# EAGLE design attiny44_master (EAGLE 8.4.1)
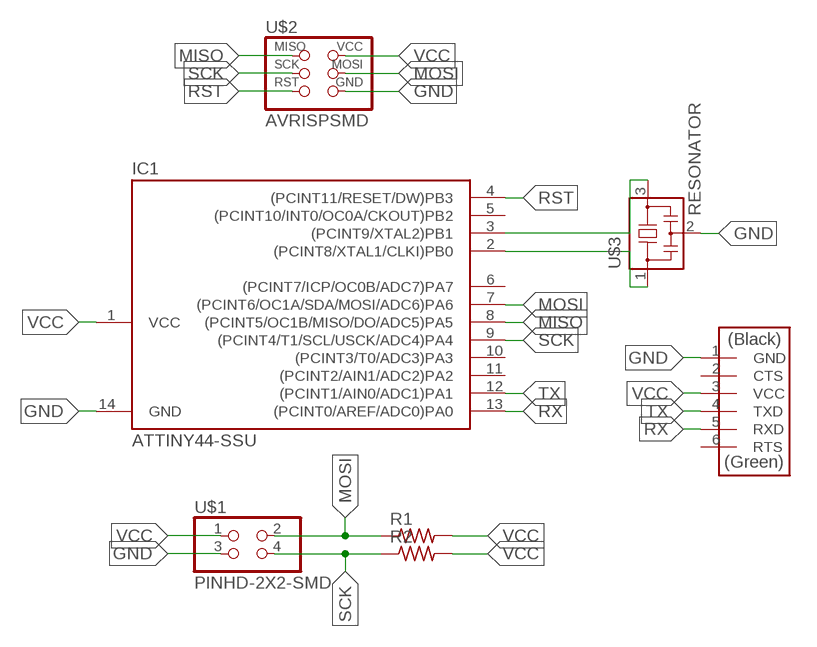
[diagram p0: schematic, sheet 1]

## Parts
IC1  ATTINY44-SSU  [SOIC14]
R1  RES-US1206FAB  [R1206FAB]
R2  RES-US1206FAB  [R1206FAB]
U$1  PINHD-2X2-SMD  [2X02SMD]
U$2  AVRISPSMD  [2X03SMD]
U$3  RESONATOR  [EFOBM]
U$4  FTDI-SMD-HEADER  [1X06SMD]

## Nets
GND: IC1.14(GND) U$1.3 U$2.6(GND) U$3.2 U$4.1(GND)
MISO: IC1.8((PCINT5/OC1B/MISO/DO/ADC5)PA5) U$2.1(MISO)
MOSI: IC1.7((PCINT6/OC1A/SDA/MOSI/ADC6)PA6) R1.1 U$1.2 U$2.4(MOSI)
N$5: IC1.3((PCINT9/XTAL2)PB1) U$3.3
N$6: IC1.2((PCINT8/XTAL1/CLKI)PB0) U$3.1
RST: IC1.4((PCINT11/RESET/DW)PB3) U$2.5(RST)
RX: IC1.13((PCINT0/AREF/ADC0)PA0) U$4.5(RXD)
SCK: IC1.9((PCINT4/T1/SCL/USCK/ADC4)PA4) R2.1 U$1.4 U$2.3(SCK)
TX: IC1.12((PCINT1/AIN0/ADC1)PA1) U$4.4(TXD)
VCC: IC1.1(VCC) R1.2 R2.2 U$1.1 U$2.2(VCC) U$4.3(VCC)
Unconnected: IC1.5((PCINT10/INT0/OC0A/CKOUT)PB2) IC1.6((PCINT7/ICP/OC0B/ADC7)PA7) IC1.10((PCINT3/T0/ADC3)PA3) IC1.11((PCINT2/AIN1/ADC2)PA2) U$4.2(CTS) U$4.6(RTS)

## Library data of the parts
IC1 = fab:ATTINY44
R1 R2 = fab:RES-US: Resistor (US Symbol)
U$1 = fab:PINHD-2X2-SMD
U$2 = fab:AVRISP
U$3 = fab:RESONATOR
U$4 = fab:FTDI-SMD-HEADER

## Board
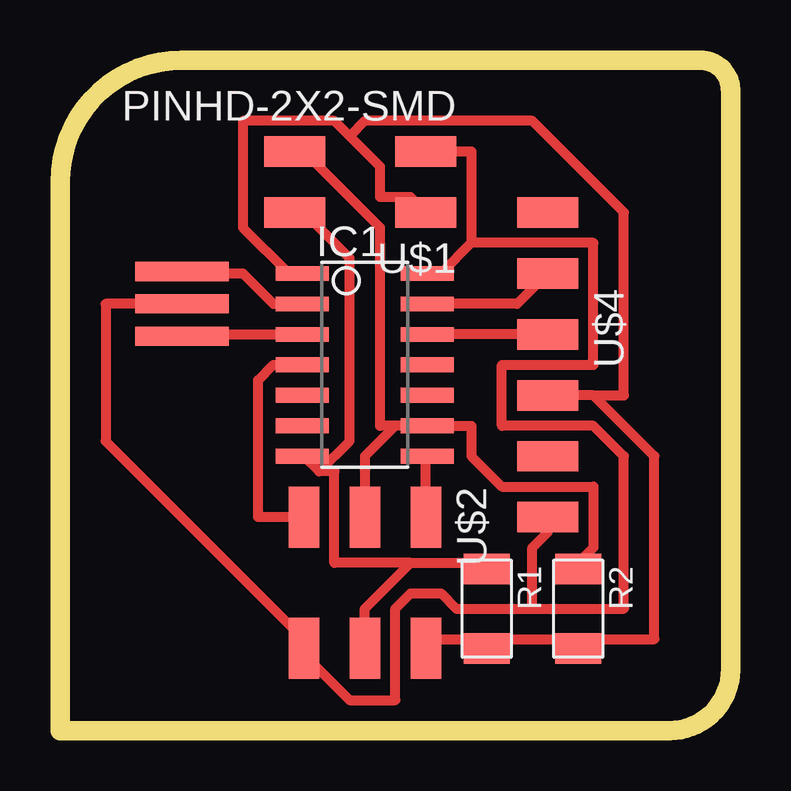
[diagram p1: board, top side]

Size 27.94 x 27.94 mm. Coordinates in mm from the lower left corner, seen from the top.
Outline: 0,22.86 arc-90 5.08,27.94 26.67,27.94 arc-90 27.94,26.67 27.94,2.54 arc-90 25.4,0 0,0 0,22.86
Copper layers (1*16): Top 0.035mm / dielectric 1.5mm / Bottom 0.035mm
Design rules "default *": minimum track width 16mil, minimum drill 0.35mm, track to track 16mil, track to pad 16mil, pad to pad 16mil, via to via 16mil, smd to smd 16mil, copper to edge 16mil, drill to drill 16mil, minimum pad ring 10mil, minimum via ring 8mil, stop-mask expansion 4mil, vias tented up to drill 0mil, thermal gap 10mil

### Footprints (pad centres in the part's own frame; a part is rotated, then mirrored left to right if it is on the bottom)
SOIC14 = smd 0.61 x 2.21: 1 -3.81,-2.603; 2 -2.54,-2.603; 3 -1.27,-2.603; 4 0,-2.603; 5 1.27,-2.603; 6 2.54,-2.603; 7 3.81,-2.603; 8 3.81,2.603; 9 2.54,2.603; 10 1.27,2.603; 11 0,2.603; 12 -1.27,2.603; 13 -2.54,2.603; 14 -3.81,2.603
R1206FAB = smd 1.27 x 1.905: 1 -1.651,0; 2 1.651,0
2X02SMD = smd 2.54 x 1.27: 1 -2.54,1.27; 2 2.92,1.27; 3 -2.54,-1.27; 4 2.92,-1.27
2X03SMD = smd 2.54 x 1.27: 1 -2.54,2.54; 2 2.92,2.54; 3 -2.54,0; 4 2.92,0; 5 -2.54,-2.54; 6 2.92,-2.54
EFOBM = smd 0.8 x 3.9: 1 -1.35,0; 2 0,0; 3 1.35,0
1X06SMD = smd 2.54 x 1.27: 1 0,6.35; 2 0,3.81; 3 0,1.27; 4 0,-1.27; 5 0,-3.81; 6 0,-6.35

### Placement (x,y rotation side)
IC1  12.7,15.24 270 top
R1  17.78,5.08 270 top
R2  21.59,5.08 270 top
U$1  12.7,22.86 180 top
U$2  12.7,6.35 270 top
U$3  5.08,17.78 270 top
U$4  20.32,15.24 180 top

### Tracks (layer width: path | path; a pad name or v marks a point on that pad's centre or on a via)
GND
  Top 0.406: 17.14,20.32 15.88,19.05 IC1.14 | 17.14,20.32 17.14,24.13 U$1.3 | U$3.2 1.9,17.78 1.9,12.07 10.16,3.81 U$2.6 10.16,3.18 12.06,1.27 13.97,1.27 13.97,5.08 14.6,5.71 15.88,5.71 16.51,5.08 19.69,5.08 | U$4.1 20.32,8.25 19.69,7.62 19.69,5.08 | 17.14,20.32 22.23,20.32 22.23,15.24 18.41,15.24 18.41,12.7 22.23,12.7 23.49,11.43 23.49,5.08 19.69,5.08
MISO
  Top 0.406: U$2.1 15.24,11.43 IC1.8
MOSI
  Top 0.406: 14.6,6.98 17.78,6.98 R1.1 | 14.6,6.98 12.7,5.08 U$2.4 | 10.79,10.79 10.16,11.43 IC1.7 | 10.79,10.79 11.43,10.79 11.43,6.98 14.6,6.98 | 10.79,10.79 12.06,12.07 12.06,19.68 10.16,21.59 U$1.2
N$5
  Top 0.406: IC1.3 5.08,16.51 U$3.3
N$6
  Top 0.406: IC1.2 8.89,17.78 7.62,19.05 5.08,19.05 U$3.1
RST
  Top 0.406: IC1.4 8.89,15.24 8.25,14.61 8.25,8.89 U$2.5
RX
  Top 0.406: IC1.13 19.05,17.78 U$4.5
SCK
  Top 0.406: R2.1 21.59,6.98 22.23,7.62 22.23,10.16 18.41,10.16 17.14,11.43 17.14,12.7 IC1.9 13.97,12.7 | 13.97,12.7 13.33,12.7 13.33,20.95 10.16,24.13 U$1.4 | U$2.3 12.7,11.43 13.97,12.7
TX
  Top 0.406: U$4.4 IC1.12
VCC
  Top 0.406: 12.06,24.76 13.33,23.5 13.33,22.22 14.6,22.22 U$1.1 | 12.06,24.76 11.43,25.4 7.62,25.4 7.62,20.95 9.52,19.05 IC1.1 | 17.78,3.81 15.24,3.81 U$2.2 | 17.78,3.81 21.59,3.81 | 17.78,3.81 R1.2 | 22.23,13.97 U$4.3 | 22.23,13.97 24.77,11.43 24.77,3.81 21.59,3.81 | 21.59,3.81 R2.2 | 12.06,24.76 12.7,25.4 19.69,25.4 23.49,21.59 23.49,13.97 22.23,13.97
